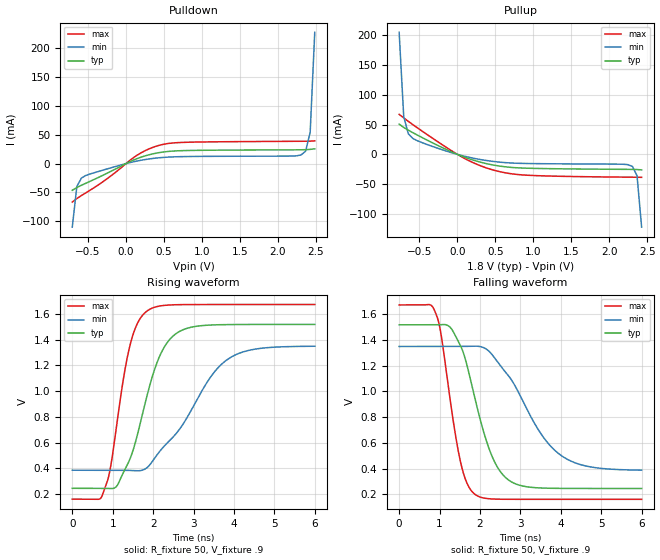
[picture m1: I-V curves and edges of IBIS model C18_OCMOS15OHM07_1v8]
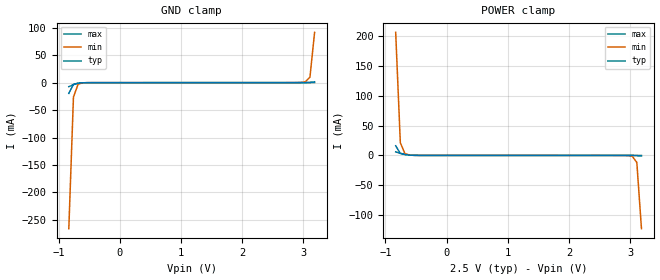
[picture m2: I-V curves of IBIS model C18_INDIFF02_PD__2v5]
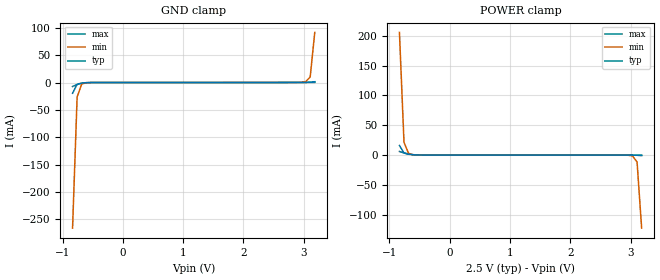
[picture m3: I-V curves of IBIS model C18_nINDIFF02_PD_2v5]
|   This file is an IBIS representation of the   |
|   Integrated Device Technology, Inc.   |
|   IDT840NT4-01I   |
|   ETHERNET & USB CLOCK GENERATOR FOR FREESCALE B4/T4 PROCESSOR SYSTEM   |
[IBIS Ver]   4.1
[File name]   840nt4_01i.ibs
[File Rev]   1.0
[Date]   21 Oct 2013
[Source]   Originated at Integrated Device Technology, Inc.
[Disclaimer]
IDT hereby grants the user of this IBIS model a non-exclusive,
nontransferable license to use this IBIS model under the following terms.
Before using this IBIS model, the user should read this license.
If the user does not accept these terms,  the IBIS model should be
returned to IDT within 30 days.
   The user is granted this license only to use the IBIS model and
is not granted rights to sell, load, rent, lease or license the IBIS
model in whole or in part, or in modified form to anyone other than
user. User may modify the IBIS model to suit its specific
applications but rights to derivative works and such modifications
shall belong to IDT.
   This IBIS model is provided on an "AS IS" basis and IDT makes
absolutely no warranty with respect to the information contained
herein. IDT DISCLAIMS AND CUSTOMER WAIVES ALL WARRANTIES, EXPRESS
OR IMPLIED, INCLUDING WARRANTIES OF MERCHANTABILITY OR FITNESS FOR
A PARTICULAR PURPOSE. The entire risk as to quality and performance
is with the Customer. ACCORDINGLY, IN NO EVENT SHALL THE COMPANY BE
LIABLE FOR ANY DAMAGES, WHETHER IN CONTRACT OR TORT,INCLUDING ANY
LOST PROFITS OR OTHER INCIDENTAL, CONSEQUENTIAL, EXEMPLARY, OR
PUNITIVE DAMAGES ARISING OUT OF THE USE OR APPLICATION OF THE IBIS
model provided in this package. Further, IDT reserves the right to
make changes without notice to any product herein to improve
reliability, function, or design. IDT does not convey any license
under patent rights or any other intellectual property rights,
including those of third parties.
   IDT is not obligated to provide maintenance or support
for the licensed IBIS model.
[Copyright] Copyright 2012 by Integrated Device Technology, Inc.
[Component]   IDT840NT4-01NLGI
[Manufacturer] Integrated Device Technology, Inc.
[Package]
|QFN48
|lead+wire   typ   min   max
R_pkg   101.2m   86.97m   132.8m
L_pkg   2.183n   1.808n   3.016n
C_pkg   0.200p   0.1726p   0.261p
[Pin] signal_name  model_name   R_pin   L_pin   C_pin
1   XTAL_IN   NC   132.8703m   3.0159n   0.261p
2   XTAL_OUT  NC   117.0583m   2.5998n   0.2305p
3   VDD   POWER   106.0039m   2.3089n   0.2093p
4   PCLK   C18_INDIFF02_PD_   95.3693m   2.029n   0.1888p
5   nPCLK   C18_nINDIFF02_PD   90.4717m   1.9001n   0.1794p
6   VDD   POWER   86.9735m   1.808n   0.1726p
7   GND   GND   87.1134m   1.8117n   0.1729p
8   PDIV_SEL  C18_INESD01_PD50   89.3523m   1.8706n   0.1772p
9   GND   GND   94.5297m   2.0069n   0.1872p
10   OE_REF   C18_INESD01_PU50   103.2053m   2.2352n   0.2039p
11   VDDO_REF  POWER   115.659m   2.563n   0.2279p
12   QREF1   C18_OCMOS15OHM07   130.3515m   2.9496n   0.2561p
13   GND   GND   132.1706m   2.9975n   0.2596p
14   OE_C   C18_INESD01_PU50   101.6661m   2.1947n   0.2009p
15   GND   GND   92.8505m   1.9627n   0.1839p
16   QC   C18_OCMOS15OHM07   87.8131m   1.8301n   0.1742p
17   VDDO_C   POWER   87.1134m   1.8117n   0.1729p
18   OE_B   C18_INESD01_PU50   88.9325m   1.8596n   0.1764p
19   VDDO_B   POWER   88.9325m   1.8596n   0.1764p
20   QB2   C18_OCMOS15OHM07   87.1134m   1.8117n   0.1729p
21   QB1   C18_OCMOS15OHM07   87.8131m   1.8301n   0.1742p
22   QB0   C18_OCMOS15OHM07   92.8505m   1.9627n   0.1839p
23   VDDO_B   POWER   101.6661m   2.1947n   0.2009p
24   GND   GND   132.1706m   2.9975n   0.2596p
25   GND   GND   130.3515m   2.9496n   0.2561p
26   GND   GND   115.659m   2.563n   0.2279p
27   QA4   C18_OCMOS15OHM07   103.2053m   2.2352n   0.2039p
28   QA3   C18_OCMOS15OHM07   94.5297m   2.0069n   0.1872p
29   QA2   C18_OCMOS15OHM07   89.3523m   1.8706n   0.1772p
30   VDDO_A   POWER   87.1134m   1.8117n   0.1729p
31   VDDO_A   POWER   86.9735m   1.808n   0.1726p
32   QA1   C18_OCMOS15OHM07   90.4717m   1.9001n   0.1794p
33   QA0   C18_OCMOS15OHM07   95.3693m   2.029n   0.1888p
34   OE_A   C18_INESD01_PU50   106.0039m   2.3089n   0.2093p
35   GND   GND   117.0583m   2.5998n   0.2305p
36   GND   GND   132.8703m   3.0159n   0.261p
37   VDD   POWER   131.6109m   2.9828n   0.2586p
38   PSELB   C18_INESD01_PD50   101.806m   2.1984n   0.2012p
39   PLL_SELA  C18_INESD01_PU50   92.7106m   1.959n   0.1837p
40   PLL_SELB  C18_INESD01_PU50   88.2329m   1.8412n   0.175p
41   GND   GND   87.2534m   1.8154n   0.1732p
42   VDDA   POWER   88.2329m   1.8412n   0.175p
43   GND   GND   88.2329m   1.8412n   0.175p
44   VDD   POWER   87.2534m   1.8154n   0.1732p
45   RESERVERD NC   88.2329m   1.8412n   0.175p
46   VDD   POWER   92.7106m   1.959n   0.1837p
47   XTAL_SEL  C18_INESD01_PD50   101.806m   2.1984n   0.2012p
48   GND   GND   131.6109m   2.9828n   0.2586p
[Diff Pin]   inv_pin   vdiff   tdelay_typ   tdelay_min  tdelay_max
4   5   0.3   NA   NA   NA
[Model Selector] C18_INDIFF02_PD_
C18_INDIFF02_PD__1v8  Buffer selection for 1v8
C18_INDIFF02_PD__2v5  Buffer selection for 2v5
C18_INDIFF02_PD__3v3  Buffer selection for 3v3
[Model Selector] C18_nINDIFF02_PD
C18_nINDIFF02_PD_1v8  Buffer selection for 1v8
C18_nINDIFF02_PD_2v5  Buffer selection for 2v5
C18_nINDIFF02_PD_3v3  Buffer selection for 3v3
[Model Selector] C18_INESD01_PD50
C18_INESD01_PD50_1v8  Buffer selection for 1v8
C18_INESD01_PD50_2v5  Buffer selection for 2v5
C18_INESD01_PD50_3v3  Buffer selection for 3v3
[Model Selector] C18_INESD01_PU50
C18_INESD01_PU50_1v8  Buffer selection for 1v8
C18_INESD01_PU50_2v5  Buffer selection for 2v5
C18_INESD01_PU50_3v3  Buffer selection for 3v3
[Model Selector] C18_OCMOS15OHM07
C18_OCMOS15OHM07_1v8  Buffer selection for 1v8
C18_OCMOS15OHM07_2v5  Buffer selection for 2v5
C18_OCMOS15OHM07_3v3  Buffer selection for 3v3
| Models and submodels in the file (11): C18_OCMOS15OHM07_1v8 (Output), C18_INDIFF02_PD__2v5 (Input), C18_nINDIFF02_PD_2v5 (Input), C18_INESD01_PD50_2v5 (Input), C18_INESD01_PU50_2v5 (Input), C18_OCMOS15OHM07_2v5 (Output), C18_INDIFF02_PD__3v3 (Input), C18_nINDIFF02_PD_3v3 (Input), C18_INESD01_PD50_3v3 (Input), C18_INESD01_PU50_3v3 (Input), C18_OCMOS15OHM07_3v3 (Output)
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[Model] C18_OCMOS15OHM07_1v8
Model_type   Output
Polarity   Non-Inverting
|   typ   min   max
C_comp   2pF   1.5pF   2.5pF
Vmeas = .9
Rref = 50
Cref = 0
Vref = .9
|   typ   min   max
[Voltage range]   1.8V   1.710V   1.890V
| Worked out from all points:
|   slope of the pulldown table from 0 to 0.27 V, typ, clamps not added: 19.2 ohm
|   slope of the pullup table from 0 to 0.27 V, typ, clamps not added: 22.7 ohm
|   rising waveform, R_fixture 50, V_fixture .9: 20-80 % time 690ps typ, 1.24ns min, 465ps max; typ from 0.245 V to 1.52 V
|   falling waveform, R_fixture 50, V_fixture .9: 20-80 % time 667ps typ, 1.12ns min, 438ps max; typ from 1.52 V to 0.245 V
[Pulldown]
|Voltage   I (typ)   I (min)   I (max)
|Note, modeling breaks down at 250mA and above.  This is well beyond the functional   |
|operating range of the device.  Should this scenario occur, catastrophic failure and   |
|possible damage to the device and/or board is of higher concern than the I-V curve   |
|behavior.  The IBIS checker will flag currents in excess of 10A with warnings.  Lines   |
|with currents in excess of 0.35 A have been commented out.  The points still remain|
|available to the user if the user desires to use them.   |
|-1.74000e+00   -1.50943e+01   -1.31205e+01   -1.74365e+01
|-1.68000e+00   -1.40541e+01   -1.23416e+01   -1.61067e+01
|-1.62000e+00   -1.30138e+01   -1.15627e+01   -1.47768e+01
|-1.56000e+00   -1.19734e+01   -1.07838e+01   -1.34468e+01
|-1.50000e+00   -1.09330e+01   -1.00049e+01   -1.21167e+01
|-1.49000e+00   -1.07596e+01   -9.87506e+00   -1.18950e+01
|-1.42977e+00   -9.71520e+00   -9.09311e+00   -1.05596e+01
|-1.36954e+00   -8.67073e+00   -8.31116e+00   -9.22415e+00
|-1.30931e+00   -7.62624e+00   -7.52921e+00   -7.88862e+00
|-1.24908e+00   -6.58176e+00   -6.74727e+00   -6.55304e+00
|-1.18885e+00   -5.53729e+00   -5.96536e+00   -5.21741e+00
|-1.12862e+00   -4.49286e+00   -5.18351e+00   -3.88178e+00
|-1.06839e+00   -3.44851e+00   -4.40173e+00   -2.54617e+00
|-1.00816e+00   -2.40428e+00   -3.62007e+00   -1.21062e+00
|-9.47931e-01   -1.36024e+00   -2.83858e+00   -2.00666e-01
|-8.87701e-01   -3.53287e-01   -2.05730e+00   -9.71251e-02
|-8.27471e-01   -8.58986e-02   -1.27635e+00   -8.30163e-02
|-7.67241e-01   -5.41249e-02   -4.95812e-01   -7.41965e-02
-707mV    -46.23mA   -110.1mA   -66.7mA
-646.8mV  -41.45mA   -39.65mA   -60.52mA
-586.6mV  -37.53mA   -25.02mA   -55.33mA
-466.1mV  -30.3mA    -17.71mA   -45.61mA
136.2mV   8.143mA    4.236mA    13.67mA
316.9mV   15.74mA    8.293mA    26.27mA
497.6mV   20.22mA    10.76mA    33.57mA
859mV     22.8mA     12.32mA    37.15mA
2.304V    23.94mA    14.91mA    38.7mA
2.365V    24.16mA    21.46mA    38.76mA
2.425V    24.67mA    54.23mA    38.92mA
2.485V    25.62mA    227.5mA    39.37mA
| 2.54540e+00   2.73534e-02   8.83756e-01   4.03212e-02
| 2.60563e+00   3.33717e-02   1.63968e+00   4.17975e-02
| 2.66586e+00   7.74372e-02   2.39576e+00   4.37305e-02
| 2.72609e+00   4.81440e-01   3.15197e+00   4.62003e-02
| 2.78632e+00   1.49109e+00   3.90831e+00   5.18397e-02
| 2.84655e+00   2.50094e+00   4.66477e+00   1.08531e-01
| 2.90678e+00   3.51095e+00   5.42134e+00   8.69076e-01
| 2.96701e+00   4.52112e+00   6.17802e+00   2.16067e+00
| 3.02724e+00   5.53143e+00   6.93480e+00   3.45247e+00
| 3.08747e+00   6.54188e+00   7.69167e+00   4.74444e+00
| 3.14770e+00   7.55246e+00   8.44865e+00   6.03659e+00
| 3.20793e+00   8.56316e+00   9.20572e+00   7.32888e+00
| 3.26816e+00   9.57397e+00   9.96289e+00   8.62132e+00
| 3.32839e+00   1.05849e+01   1.07202e+01   9.91389e+00
| 3.38862e+00   1.15959e+01   1.14775e+01   1.12066e+01
| 3.44885e+00   1.26071e+01   1.22350e+01   1.24994e+01
| 3.50908e+00   1.36183e+01   1.29925e+01   1.37923e+01
| 3.56931e+00   1.46297e+01   1.37502e+01   1.50854e+01
| 3.62954e+00   1.56411e+01   1.45080e+01   1.63786e+01
| 3.68977e+00   1.66527e+01   1.52659e+01   1.76718e+01
| 3.75000e+00   1.76644e+01   1.60239e+01   1.89652e+01
| 3.76000e+00   1.78324e+01   1.61497e+01   1.91800e+01
| 3.72800e+00   1.72949e+01   1.57470e+01   1.84928e+01
| 3.69600e+00   1.67574e+01   1.53443e+01   1.78056e+01
| 3.66400e+00   1.62199e+01   1.49416e+01   1.71185e+01
| 3.63200e+00   1.56825e+01   1.45389e+01   1.64314e+01
| 3.60000e+00   1.51450e+01   1.41363e+01   1.57443e+01
[Pullup]
|Voltage   I (typ)   I (min)   I (max)
|Note, modeling breaks down at 250mA and above.  This is well beyond the functional   |
|operating range of the device.  Should this scenario occur, catastrophic failure and   |
|possible damage to the device and/or board is of higher concern than the I-V curve   |
|behavior.  The IBIS checker will flag currents in excess of 10A with warnings.  Lines   |
|with currents in excess of 0.35 A have been commented out.  The points still remain|
|available to the user if the user desires to use them.   |
|-1.74000e+00   1.41997e+01   1.23010e+01   1.64587e+01
|-1.68000e+00   1.31899e+01   1.15443e+01   1.51679e+01
|-1.62000e+00   1.21803e+01   1.07878e+01   1.38773e+01
|-1.56000e+00   1.11707e+01   1.00315e+01   1.25867e+01
|-1.50000e+00   1.01613e+01   9.27523e+00   1.12963e+01
|-1.49000e+00   9.99307e+00   9.14921e+00   1.10812e+01
|-1.42977e+00   8.97991e+00   8.39020e+00   9.78597e+00
|-1.36954e+00   7.96687e+00   7.63131e+00   8.49082e+00
|-1.30931e+00   6.95393e+00   6.87253e+00   7.19576e+00
|-1.24908e+00   5.94109e+00   6.11385e+00   5.90080e+00
|-1.18885e+00   4.92835e+00   5.35527e+00   4.60591e+00
|-1.12862e+00   3.91571e+00   4.59679e+00   3.31112e+00
|-1.06839e+00   2.90315e+00   3.83840e+00   2.01640e+00
|-1.00816e+00   1.89069e+00   3.08010e+00   7.21769e-01
|-9.47931e-01   8.78329e-01   2.32189e+00   1.23173e-01
|-8.87701e-01   1.65861e-01   1.56378e+00   8.13247e-02
|-8.27471e-01   6.54918e-02   8.05762e-01   7.31858e-02
-767.2mV  50.77mA    204.6mA    67.04mA
-707mV    45.16mA    63.38mA    61.14mA
-646.8mV  40.63mA    34.58mA    55.39mA
-586.6mV  36.37mA    26.69mA    49.82mA
75.98mV   -3.828mA   -2.537mA   -5.57mA
316.9mV   -13.5mA    -8.961mA   -19.75mA
557.8mV   -19.63mA   -13.03mA   -29mA
979.4mV   -23.37mA   -15.4mA    -35.3mA
2.244V    -25.12mA   -17.19mA   -38.18mA
2.304V    -25.2mA    -20.2mA    -38.25mA
2.365V    -25.4mA    -35.93mA   -38.33mA
2.425V    -25.96mA   -122mA     -38.47mA
| 2.48517e+00   -2.74001e-02   -5.87391e-01   -3.88904e-02
| 2.54540e+00   -3.09996e-02   -1.36663e+00   -4.01601e-02
| 2.60563e+00   -4.57940e-02   -2.14645e+00   -4.31057e-02
| 2.66586e+00   -1.62932e-01   -2.92672e+00   -4.80619e-02
| 2.72609e+00   -9.56840e-01   -3.70734e+00   -5.50416e-02
| 2.78632e+00   -1.99958e+00   -4.48823e+00   -7.02072e-02
| 2.84655e+00   -3.04277e+00   -5.26933e+00   -2.22318e-01
| 2.90678e+00   -4.08632e+00   -6.05060e+00   -1.36885e+00
| 2.96701e+00   -5.13013e+00   -6.83201e+00   -2.70389e+00
| 3.02724e+00   -6.17414e+00   -7.61352e+00   -4.03920e+00
| 3.08747e+00   -7.21830e+00   -8.39512e+00   -5.37469e+00
| 3.14770e+00   -8.26257e+00   -9.17678e+00   -6.71030e+00
| 3.20793e+00   -9.30692e+00   -9.95849e+00   -8.04598e+00
| 3.26816e+00   -1.03513e+01   -1.07402e+01   -9.38167e+00
| 3.32839e+00   -1.13957e+01   -1.15220e+01   -1.07174e+01
| 3.38862e+00   -1.24402e+01   -1.23038e+01   -1.20530e+01
| 3.44885e+00   -1.34846e+01   -1.30855e+01   -1.33886e+01
| 3.50908e+00   -1.45289e+01   -1.38673e+01   -1.47241e+01
| 3.56931e+00   -1.55733e+01   -1.46491e+01   -1.60595e+01
| 3.62954e+00   -1.66176e+01   -1.54308e+01   -1.73949e+01
| 3.68977e+00   -1.76618e+01   -1.62125e+01   -1.87301e+01
| 3.75000e+00   -1.87060e+01   -1.69942e+01   -2.00652e+01
| 3.76000e+00   -1.88793e+01   -1.71242e+01   -2.02869e+01
| 3.72800e+00   -1.83246e+01   -1.67086e+01   -1.95775e+01
| 3.69600e+00   -1.77698e+01   -1.62933e+01   -1.88682e+01
| 3.66400e+00   -1.72150e+01   -1.58780e+01   -1.81588e+01
| 3.63200e+00   -1.66602e+01   -1.54627e+01   -1.74494e+01
| 3.60000e+00   -1.61054e+01   -1.50474e+01   -1.67399e+01
[Ramp]
|   typ   min   max
dV/dt_r   0.765/0.692n   0.58/1.251n   0.907/0.464n
dV/dt_f   0.765/0.667n   0.578/1.122n   0.909/0.438n
R_load =   50.0000
[Rising Waveform]
R_fixture = 50
V_fixture = .9   |Vcc_typ
V_fixture_min = .855 |Vcc_min
V_fixture_max = .945 |Vcc_max
C_fixture = 0.0p
| Time   typ   min   max
0s        244.7mV    385mV      160.3mV
738.7ps   244.8mV    385mV      186.8mV
936.9ps   242.5mV    385.1mV    391.7mV
1.417ns   464.9mV    383.8mV    1.341V
1.832ns   942.2mV    400.9mV    1.617V
2.234ns   1.318V     558.1mV    1.664V
2.727ns   1.474V     736.3mV    1.671V
3.429ns   1.513V     1.112V     1.672V
3.922ns   1.516V     1.262V     1.672V
6ns       1.517V     1.348V     1.672V
[Falling Waveform]
R_fixture = 50
V_fixture = .9   |Vcc_typ
V_fixture_min = .855 |Vcc_min
V_fixture_max = .945 |Vcc_max
C_fixture = 0.0p
| Time   typ   min   max
0s        1.517V     1.349V     1.672V
906.9ps   1.517V     1.349V     1.606V
1.039ns   1.519V     1.349V     1.439V
1.508ns   1.362V     1.349V     467.2mV
1.868ns   954.9mV    1.352V     201.1mV
2.312ns   485.1mV    1.281V     162.8mV
2.793ns   293.6mV    1.083V     160.4mV
3.489ns   248.7mV    679.3mV    160.3mV
4.024ns   245.3mV    497.9mV    160.3mV
6ns       244.7mV    387.1mV    160.3mV
[Model] C18_INDIFF02_PD__2v5
Model_type   Input
Polarity   Non-Inverting
Vinl = 0.7V
Vinh = 1.7V
|   typ   min   max
C_comp   2pF   1.5pF   2.5pF
|   typ   min   max
[Voltage range]   2.5V   2.375V   2.625V
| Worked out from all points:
|   GND clamp passes 1 mA (typ) near -0.68 V on its own axis
|   POWER clamp passes 1 mA (typ) near -0.65 V on its own axis
[GND_clamp]
|Voltage   I (typ)   I (min)   I (max)
|Note, modeling breaks down at 250mA and above.  This is well beyond the functional   |
|operating range of the device.  Should this scenario occur, catastrophic failure and   |
|possible damage to the device and/or board is of higher concern than the I-V curve   |
|behavior.  The IBIS checker will flag currents in excess of 10A with warnings.  Lines   |
|with currents in excess of 0.35 A have been commented out.  The points still remain|
|available to the user if the user desires to use them.   |
|-2.50000e+00   -1.17751e+01   -1.02956e+01   -1.42771e+01
|-2.42424e+00   -1.12273e+01   -9.83975e+00   -1.35770e+01
|-2.34848e+00   -1.06795e+01   -9.38384e+00   -1.28768e+01
|-2.27273e+00   -1.01317e+01   -8.92789e+00   -1.21765e+01
|-2.19697e+00   -9.58377e+00   -8.47190e+00   -1.14762e+01
|-2.12121e+00   -9.03579e+00   -8.01587e+00   -1.07757e+01
|-2.04545e+00   -8.48775e+00   -7.55981e+00   -1.00751e+01
|-1.96970e+00   -7.93965e+00   -7.10372e+00   -9.37444e+00
|-1.89394e+00   -7.39150e+00   -6.64760e+00   -8.67368e+00
|-1.81818e+00   -6.84330e+00   -6.19147e+00   -7.97283e+00
|-1.74242e+00   -6.29506e+00   -5.73532e+00   -7.27190e+00
|-1.66667e+00   -5.74679e+00   -5.27916e+00   -6.57089e+00
|-1.59091e+00   -5.19849e+00   -4.82301e+00   -5.86980e+00
|-1.51515e+00   -4.65019e+00   -4.36687e+00   -5.16866e+00
|-1.43939e+00   -4.10189e+00   -3.91076e+00   -4.46747e+00
|-1.36364e+00   -3.55361e+00   -3.45470e+00   -3.76626e+00
|-1.28788e+00   -3.00539e+00   -2.99869e+00   -3.06504e+00
|-1.21212e+00   -2.45724e+00   -2.54278e+00   -2.36385e+00
|-1.13636e+00   -1.90921e+00   -2.08698e+00   -1.66274e+00
|-1.06061e+00   -1.36135e+00   -1.63133e+00   -9.61760e-01
|-9.84848e-01   -8.13726e-01   -1.17589e+00   -2.61004e-01
|-9.09091e-01   -2.66435e-01   -7.20720e-01   -1.76899e-02
-833.3mV  -19.53mA   -265.9mA   -7.283mA
-757.6mV  -3.155mA   -26.29mA   -3.549mA
-681.8mV  -925uA     -2.786mA   -1.24mA
-530.3mV  -53.72uA   -66.97uA   -51.38uA
2.803V    56.14uA    61.7uA     59.51uA
3.03V     157.7uA    1.578mA    66.02uA
3.106V    515.4uA    10.06mA    89.24uA
3.182V    1.393mA    91.56mA    263.3uA
| 3.25758e+00   3.36773e-03   7.21068e-01   9.40408e-04
| 3.33333e+00   1.60551e-02   1.60184e+00   2.31196e-03
| 3.40909e+00   2.04586e-01   2.48282e+00   4.29776e-03
| 3.48485e+00   1.20199e+00   3.36399e+00   7.21000e-03
| 3.56061e+00   2.26047e+00   4.24533e+00   2.70381e-02
| 3.63636e+00   3.31917e+00   5.12682e+00   5.94881e-01
| 3.71212e+00   4.37807e+00   6.00846e+00   1.94865e+00
| 3.78788e+00   5.43715e+00   6.89024e+00   3.30267e+00
| 3.86364e+00   6.49639e+00   7.77215e+00   4.65692e+00
| 3.93939e+00   7.55578e+00   8.65419e+00   6.01137e+00
| 4.01515e+00   8.61532e+00   9.53637e+00   7.36599e+00
| 4.09091e+00   9.67500e+00   1.04187e+01   8.72078e+00
| 4.16667e+00   1.07348e+01   1.13011e+01   1.00757e+01
| 4.24242e+00   1.17948e+01   1.21837e+01   1.14308e+01
| 4.31818e+00   1.28548e+01   1.30664e+01   1.27860e+01
| 4.39394e+00   1.39150e+01   1.39492e+01   1.41414e+01
| 4.46970e+00   1.49754e+01   1.48323e+01   1.54968e+01
| 4.54545e+00   1.60359e+01   1.57154e+01   1.68524e+01
| 4.62121e+00   1.70965e+01   1.65988e+01   1.82082e+01
| 4.69697e+00   1.81574e+01   1.74824e+01   1.95641e+01
| 4.77273e+00   1.92184e+01   1.83661e+01   2.09201e+01
| 4.84848e+00   2.02795e+01   1.92502e+01   2.22763e+01
| 4.92424e+00   2.13409e+01   2.01344e+01   2.36326e+01
| 5.00000e+00   2.24025e+01   2.10190e+01   2.49892e+01
[Power_clamp]
|Voltage   I (typ)   I (min)   I (max)
|Note, modeling breaks down at 250mA and above.  This is well beyond the functional   |
|operating range of the device.  Should this scenario occur, catastrophic failure and   |
|possible damage to the device and/or board is of higher concern than the I-V curve   |
|behavior.  The IBIS checker will flag currents in excess of 10A with warnings.  Lines   |
|with currents in excess of 0.35 A have been commented out.  The points still remain|
|available to the user if the user desires to use them.   |
|-2.50000e+00   2.24025e+01   1.95596e+01   2.72279e+01
|-2.42424e+00   2.13409e+01   1.86755e+01   2.58710e+01
|-2.34848e+00   2.02795e+01   1.77917e+01   2.45144e+01
|-2.27273e+00   1.92184e+01   1.69080e+01   2.31579e+01
|-2.19697e+00   1.81574e+01   1.60246e+01   2.18016e+01
|-2.12121e+00   1.70965e+01   1.51413e+01   2.04455e+01
|-2.04545e+00   1.60359e+01   1.42583e+01   1.90895e+01
|-1.96970e+00   1.49754e+01   1.33754e+01   1.77337e+01
|-1.89394e+00   1.39150e+01   1.24926e+01   1.63780e+01
|-1.81818e+00   1.28548e+01   1.16100e+01   1.50224e+01
|-1.74242e+00   1.17948e+01   1.07275e+01   1.36670e+01
|-1.66667e+00   1.07348e+01   9.84516e+00   1.23117e+01
|-1.59091e+00   9.67500e+00   8.96294e+00   1.09565e+01
|-1.51515e+00   8.61532e+00   8.08085e+00   9.60148e+00
|-1.43939e+00   7.55578e+00   7.19889e+00   8.24659e+00
|-1.36364e+00   6.49639e+00   6.31706e+00   6.89185e+00
|-1.28788e+00   5.43715e+00   5.43537e+00   5.53729e+00
|-1.21212e+00   4.37807e+00   4.55383e+00   4.18291e+00
|-1.13636e+00   3.31917e+00   3.67244e+00   2.82874e+00
|-1.06061e+00   2.26047e+00   2.79121e+00   1.47480e+00
|-9.84848e-01   1.20199e+00   1.91016e+00   1.95515e-01
|-9.09091e-01   2.04586e-01   1.02931e+00   1.34664e-02
-833.3mV  16.06mA    205.8mA    5.965mA
-757.6mV  3.368mA    21.21mA    3.538mA
-681.8mV  1.393mA    2.864mA    1.756mA
-606.1mV  515.4uA    588.8uA    625.4uA
-454.5mV  72.76uA    70.8uA     75.22uA
2.879V    -8.33uA    -39.85uA   -5.39uA
3.03V     -53.72uA   -1.341mA   -9.307uA
3.106V    -239.1uA   -11.72mA   -19.64uA
3.182V    -925uA     -122.5mA   -93.12uA
| 3.25758e+00   -3.15473e-03   -5.61496e-01   -4.94368e-04
| 3.33333e+00   -1.95321e-02   -1.01654e+00   -1.88092e-03
| 3.40909e+00   -2.66435e-01   -1.47190e+00   -4.68973e-03
| 3.48485e+00   -8.13726e-01   -1.92748e+00   -9.15894e-03
| 3.56061e+00   -1.36135e+00   -2.38323e+00   -3.57878e-02
| 3.63636e+00   -1.90921e+00   -2.83911e+00   -5.06236e-01
| 3.71212e+00   -2.45724e+00   -3.29509e+00   -1.20708e+00
| 3.78788e+00   -3.00539e+00   -3.75113e+00   -1.90812e+00
| 3.86364e+00   -3.55361e+00   -4.20723e+00   -2.60926e+00
| 3.93939e+00   -4.10189e+00   -4.66336e+00   -3.31047e+00
| 4.01515e+00   -4.65019e+00   -5.11951e+00   -4.01169e+00
| 4.09091e+00   -5.19849e+00   -5.57566e+00   -4.71289e+00
| 4.16667e+00   -5.74679e+00   -6.03181e+00   -5.41407e+00
| 4.24242e+00   -6.29506e+00   -6.48796e+00   -6.11519e+00
| 4.31818e+00   -6.84330e+00   -6.94408e+00   -6.81625e+00
| 4.39394e+00   -7.39150e+00   -7.40018e+00   -7.51723e+00
| 4.46970e+00   -7.93965e+00   -7.85625e+00   -8.21814e+00
| 4.54545e+00   -8.48775e+00   -8.31229e+00   -8.91896e+00
| 4.62121e+00   -9.03579e+00   -8.76829e+00   -9.61969e+00
| 4.69697e+00   -9.58377e+00   -9.22426e+00   -1.03203e+01
| 4.77273e+00   -1.01317e+01   -9.68018e+00   -1.10209e+01
| 4.84848e+00   -1.06795e+01   -1.01361e+01   -1.17213e+01
| 4.92424e+00   -1.12273e+01   -1.05919e+01   -1.24217e+01
| 5.00000e+00   -1.17751e+01   -1.10477e+01   -1.31219e+01
[Model] C18_nINDIFF02_PD_2v5
Model_type   Input
Polarity   Non-Inverting
Vinl = 0.7V
Vinh = 1.7V
|   typ   min   max
C_comp   2pF   1.5pF   2.5pF
|   typ   min   max
[Voltage range]   2.5V   2.375V   2.625V
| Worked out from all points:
|   GND clamp passes 1 mA (typ) near -0.68 V on its own axis
|   POWER clamp passes 1 mA (typ) near -0.65 V on its own axis
[GND_clamp]
|Voltage   I (typ)   I (min)   I (max)
|Note, modeling breaks down at 250mA and above.  This is well beyond the functional   |
|operating range of the device.  Should this scenario occur, catastrophic failure and   |
|possible damage to the device and/or board is of higher concern than the I-V curve   |
|behavior.  The IBIS checker will flag currents in excess of 10A with warnings.  Lines   |
|with currents in excess of 0.35 A have been commented out.  The points still remain|
|available to the user if the user desires to use them.   |
|-2.50000e+00   -1.17752e+01   -1.02957e+01   -1.42772e+01
|-2.42424e+00   -1.12274e+01   -9.83984e+00   -1.35771e+01
|-2.34848e+00   -1.06796e+01   -9.38392e+00   -1.28769e+01
|-2.27273e+00   -1.01318e+01   -8.92797e+00   -1.21767e+01
|-2.19697e+00   -9.58387e+00   -8.47198e+00   -1.14763e+01
|-2.12121e+00   -9.03588e+00   -8.01595e+00   -1.07758e+01
|-2.04545e+00   -8.48784e+00   -7.55989e+00   -1.00752e+01
|-1.96970e+00   -7.93974e+00   -7.10380e+00   -9.37454e+00
|-1.89394e+00   -7.39159e+00   -6.64768e+00   -8.67378e+00
|-1.81818e+00   -6.84339e+00   -6.19154e+00   -7.97293e+00
|-1.74242e+00   -6.29514e+00   -5.73539e+00   -7.27199e+00
|-1.66667e+00   -5.74687e+00   -5.27924e+00   -6.57098e+00
|-1.59091e+00   -5.19857e+00   -4.82308e+00   -5.86989e+00
|-1.51515e+00   -4.65027e+00   -4.36695e+00   -5.16875e+00
|-1.43939e+00   -4.10197e+00   -3.91083e+00   -4.46756e+00
|-1.36364e+00   -3.55369e+00   -3.45477e+00   -3.76634e+00
|-1.28788e+00   -3.00546e+00   -2.99876e+00   -3.06512e+00
|-1.21212e+00   -2.45731e+00   -2.54285e+00   -2.36393e+00
|-1.13636e+00   -1.90928e+00   -2.08704e+00   -1.66282e+00
|-1.06061e+00   -1.36142e+00   -1.63139e+00   -9.61838e-01
|-9.84848e-01   -8.13796e-01   -1.17595e+00   -2.61081e-01
|-9.09091e-01   -2.66503e-01   -7.20781e-01   -1.77649e-02
-833.3mV  -19.6mA    -266mA     -7.357mA
-757.6mV  -3.22mA    -26.35mA   -3.621mA
-681.8mV  -988.6uA   -2.843mA   -1.31mA
-530.3mV  -114.3uA   -121.3uA   -118.4uA
2.803V    62.2uA     69.71uA    63.29uA
3.03V     168.3uA    1.59mA     74.62uA
3.106V    527.5uA    10.07mA    99.45uA
3.182V    1.407mA    91.57mA    275.1uA
| 3.25758e+00   3.38287e-03   7.21084e-01   9.53838e-04
| 3.33333e+00   1.60717e-02   1.60186e+00   2.32699e-03
| 3.40909e+00   2.04604e-01   2.48284e+00   4.31441e-03
| 3.48485e+00   1.20201e+00   3.36401e+00   7.22826e-03
| 3.56061e+00   2.26050e+00   4.24535e+00   2.70580e-02
| 3.63636e+00   3.31920e+00   5.12684e+00   5.94903e-01
| 3.71212e+00   4.37810e+00   6.00848e+00   1.94867e+00
| 3.78788e+00   5.43717e+00   6.89026e+00   3.30270e+00
| 3.86364e+00   6.49642e+00   7.77218e+00   4.65695e+00
| 3.93939e+00   7.55581e+00   8.65422e+00   6.01139e+00
| 4.01515e+00   8.61535e+00   9.53640e+00   7.36602e+00
| 4.09091e+00   9.67503e+00   1.04187e+01   8.72081e+00
| 4.16667e+00   1.07348e+01   1.13011e+01   1.00758e+01
| 4.24242e+00   1.17948e+01   1.21837e+01   1.14308e+01
| 4.31818e+00   1.28549e+01   1.30664e+01   1.27860e+01
| 4.39394e+00   1.39151e+01   1.39493e+01   1.41414e+01
| 4.46970e+00   1.49754e+01   1.48323e+01   1.54969e+01
| 4.54545e+00   1.60359e+01   1.57155e+01   1.68525e+01
| 4.62121e+00   1.70966e+01   1.65988e+01   1.82082e+01
| 4.69697e+00   1.81574e+01   1.74824e+01   1.95641e+01
| 4.77273e+00   1.92184e+01   1.83662e+01   2.09201e+01
| 4.84848e+00   2.02796e+01   1.92502e+01   2.22763e+01
| 4.92424e+00   2.13410e+01   2.01345e+01   2.36327e+01
| 5.00000e+00   2.24026e+01   2.10190e+01   2.49892e+01
[Power_clamp]
|Voltage   I (typ)   I (min)   I (max)
|Note, modeling breaks down at 250mA and above.  This is well beyond the functional   |
|operating range of the device.  Should this scenario occur, catastrophic failure and   |
|possible damage to the device and/or board is of higher concern than the I-V curve   |
|behavior.  The IBIS checker will flag currents in excess of 10A with warnings.  Lines   |
|with currents in excess of 0.35 A have been commented out.  The points still remain|
|available to the user if the user desires to use them.   |
|-2.50000e+00   2.24026e+01   1.95597e+01   2.72279e+01
|-2.42424e+00   2.13410e+01   1.86756e+01   2.58711e+01
|-2.34848e+00   2.02796e+01   1.77917e+01   2.45144e+01
|-2.27273e+00   1.92184e+01   1.69081e+01   2.31579e+01
|-2.19697e+00   1.81574e+01   1.60246e+01   2.18016e+01
|-2.12121e+00   1.70966e+01   1.51414e+01   2.04455e+01
|-2.04545e+00   1.60359e+01   1.42583e+01   1.90895e+01
|-1.96970e+00   1.49754e+01   1.33754e+01   1.77337e+01
|-1.89394e+00   1.39151e+01   1.24926e+01   1.63780e+01
|-1.81818e+00   1.28549e+01   1.16100e+01   1.50224e+01
|-1.74242e+00   1.17948e+01   1.07275e+01   1.36670e+01
|-1.66667e+00   1.07348e+01   9.84519e+00   1.23117e+01
|-1.59091e+00   9.67503e+00   8.96297e+00   1.09565e+01
|-1.51515e+00   8.61535e+00   8.08088e+00   9.60151e+00
|-1.43939e+00   7.55581e+00   7.19892e+00   8.24662e+00
|-1.36364e+00   6.49642e+00   6.31709e+00   6.89188e+00
|-1.28788e+00   5.43717e+00   5.43540e+00   5.53732e+00
|-1.21212e+00   4.37810e+00   4.55385e+00   4.18293e+00
|-1.13636e+00   3.31920e+00   3.67246e+00   2.82876e+00
|-1.06061e+00   2.26050e+00   2.79123e+00   1.47482e+00
|-9.84848e-01   1.20201e+00   1.91018e+00   1.95536e-01
|-9.09091e-01   2.04604e-01   1.02933e+00   1.34857e-02
-833.3mV  16.07mA    205.9mA    5.983mA
-757.6mV  3.383mA    21.22mA    3.554mA
-681.8mV  1.407mA    2.877mA    1.771mA
-606.1mV  527.5uA    600.2uA    638.2uA
-454.5mV  81.85uA    79.3uA     84.87uA
2.879V    -65.87uA   -93.69uA   -66.51uA
3.03V     -114.3uA   -1.397mA   -73.64uA
3.106V    -301.2uA   -11.78mA   -85.59uA
3.182V    -988.6uA   -122.6mA   -160.7uA
